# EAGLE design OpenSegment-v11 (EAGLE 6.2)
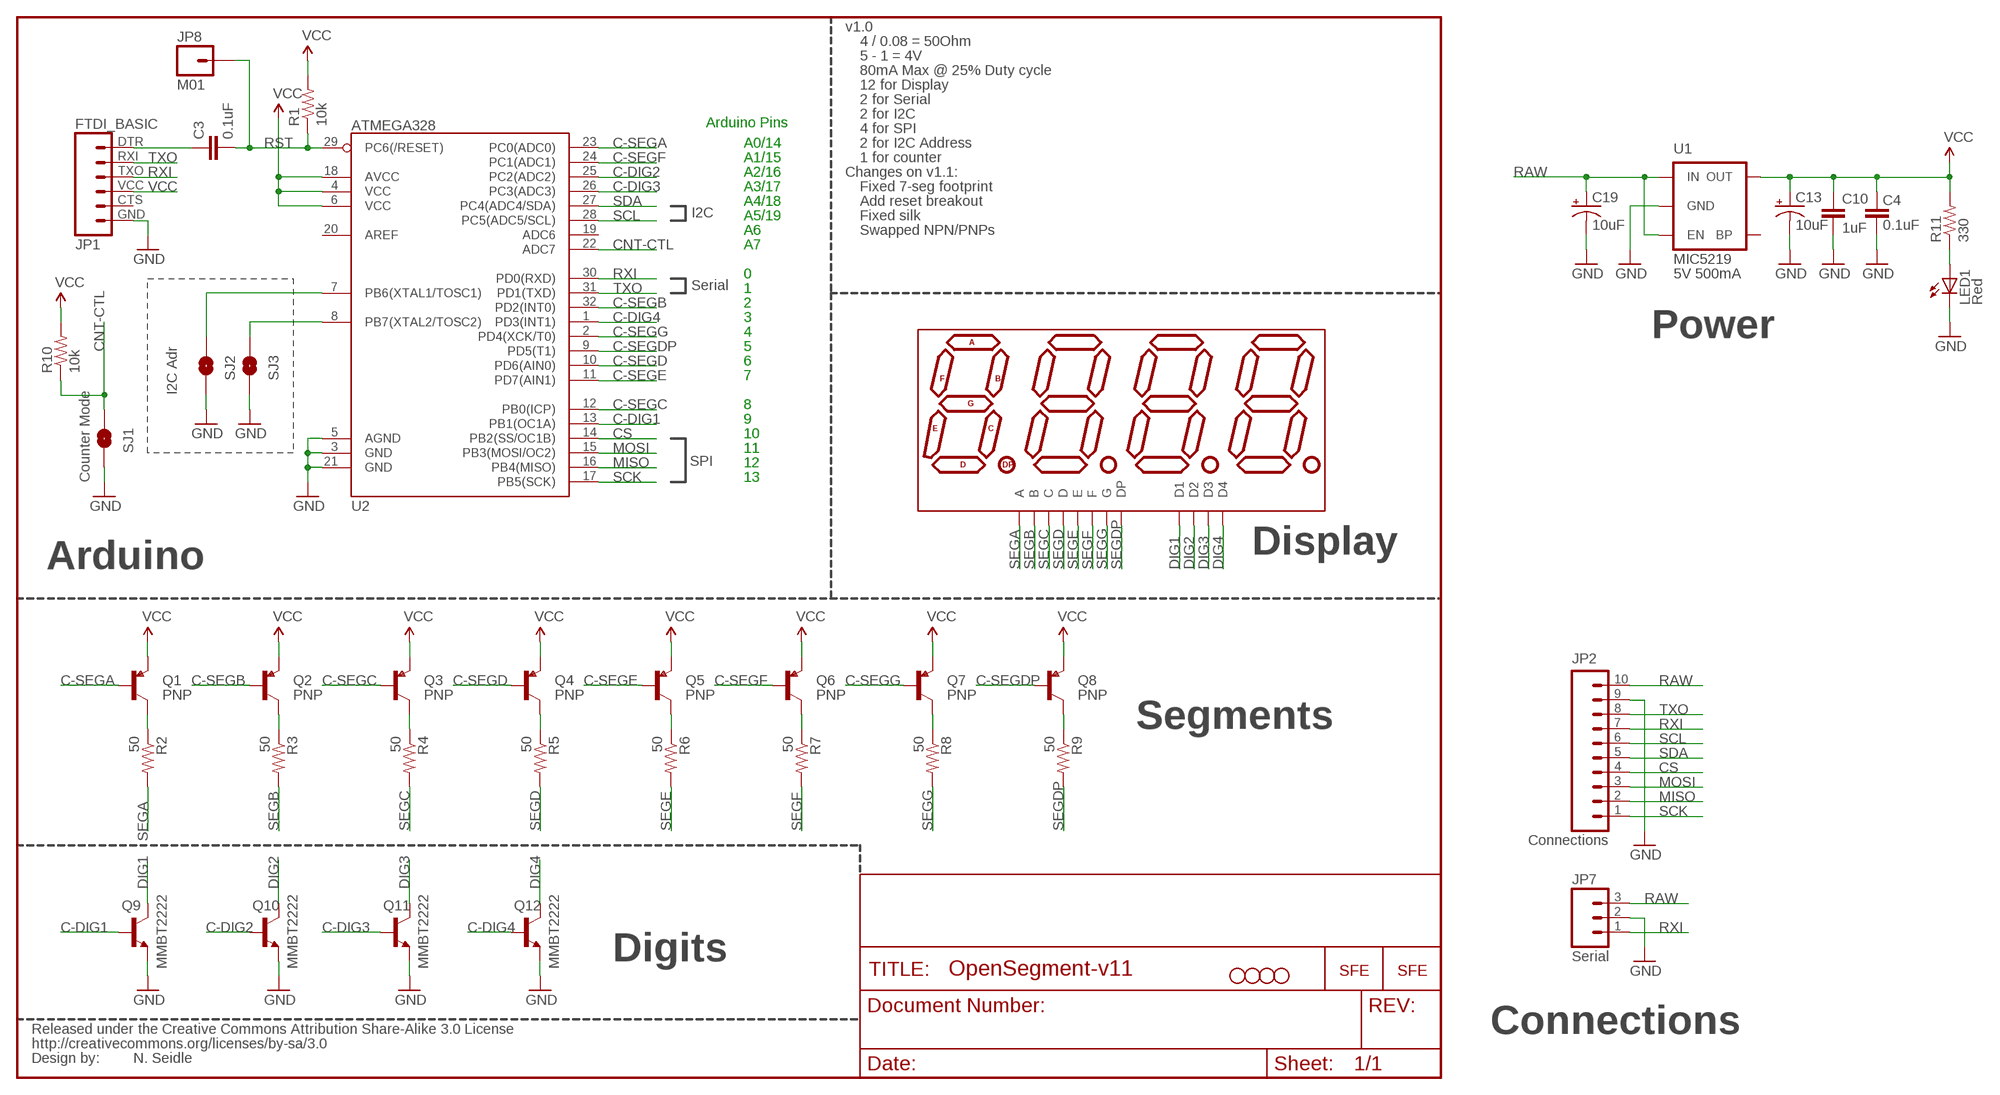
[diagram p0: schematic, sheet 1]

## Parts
C3  0.1uF  CAP0402-CAP  [0402-CAP]
C4  0.1uF  CAP0402-CAP  [0402-CAP]
C10  1uF  CAP0402-CAP  [0402-CAP]
C13  10uF  CAP_POL1206  [EIA3216]
C19  10uF  CAP_POL1206  [EIA3216]
JP1  FTDI_BASIC  FTDI_BASICPTH  [FTDI_BASIC]
JP2  Connections  M10"  [1X10]
JP3  STAND-OFF  [STAND-OFF]
JP4  STAND-OFF  [STAND-OFF]
JP5  STAND-OFF  [STAND-OFF]
JP6  STAND-OFF  [STAND-OFF]
JP7  Serial  M03  [JST-3-SMD]
JP8  M01  M01PTH  [1X01]
LED1  Red  LED0603  [LED-0603]
Q1  PNP  TRANSISTOR_PNPSMD  [SOT23-3]
Q2  PNP  TRANSISTOR_PNPSMD  [SOT23-3]
Q3  PNP  TRANSISTOR_PNPSMD  [SOT23-3]
Q4  PNP  TRANSISTOR_PNPSMD  [SOT23-3]
Q5  PNP  TRANSISTOR_PNPSMD  [SOT23-3]
Q6  PNP  TRANSISTOR_PNPSMD  [SOT23-3]
Q7  PNP  TRANSISTOR_PNPSMD  [SOT23-3]
Q8  PNP  TRANSISTOR_PNPSMD  [SOT23-3]
Q9  MMBT2222  TRANSISTOR_NPNSOT23-3  [SOT23-3]
Q10  MMBT2222  TRANSISTOR_NPNSOT23-3  [SOT23-3]
Q11  MMBT2222  TRANSISTOR_NPNSOT23-3  [SOT23-3]
Q12  MMBT2222  TRANSISTOR_NPNSOT23-3  [SOT23-3]
R1  10k  RESISTOR0402-RES  [0402-RES]
R2  50  RESISTOR0402-RES  [0402-RES]
R3  50  RESISTOR0402-RES  [0402-RES]
R4  50  RESISTOR0402-RES  [0402-RES]
R5  50  RESISTOR0402-RES  [0402-RES]
R6  50  RESISTOR0402-RES  [0402-RES]
R7  50  RESISTOR0402-RES  [0402-RES]
R8  50  RESISTOR0402-RES  [0402-RES]
R9  50  RESISTOR0402-RES  [0402-RES]
R10  10k  RESISTOR0402-RES  [0402-RES]
R11  330  RESISTOR0402-RES  [0402-RES]
SJ1  Counter Ctl  SOLDERJUMPERNO  [SJ_2S-NO]
SJ2  Counter Ctl  SOLDERJUMPERNO  [SJ_2S-NO]
SJ3  Counter Ctl  SOLDERJUMPERNO  [SJ_2S-NO]
U1  MIC5219  V_REG_LDOSMD  [SOT23-5]
U2  ATMEGA328  ATMEGA168  [TQFP32-08]
U3  7-SEGMENT-4DIGIT-COUNTERPTH  [7-SEGMENT-4DIGIT-COUNTER]
U$2  LOGO-SFESK  [SFE-LOGO-FLAME]
U$3  CREATIVE_COMMONS  [CREATIVE_COMMONS]
U$7  LOGO-SFENW2  [SFE-NEW-WEB]

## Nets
C-DIG1: Q9.1(B) U2.13(PB1(OC1A))
C-DIG2: Q10.1(B) U2.25(PC2(ADC2))
C-DIG3: Q11.1(B) U2.26(PC3(ADC3))
C-DIG4: Q12.1(B) U2.1(PD3(INT1))
C-SEGA: Q1.1(B) U2.23(PC0(ADC0))
C-SEGB: Q2.1(B) U2.32(PD2(INT0))
C-SEGC: Q3.1(B) U2.12(PB0(ICP))
C-SEGD: Q4.1(B) U2.10(PD6(AIN0))
C-SEGDP: Q8.1(B) U2.9(PD5(T1))
C-SEGE: Q5.1(B) U2.11(PD7(AIN1))
C-SEGF: Q6.1(B) U2.24(PC1(ADC1))
C-SEGG: Q7.1(B) U2.2(PD4(XCK/T0))
CNT-CTL: R10.1 SJ1.1 U2.22(ADC7)
CS: JP2.4 U2.14(PB2(SS/OC1B))
DIG1: Q9.3(C) U3.12(D1)
DIG2: Q10.3(C) U3.9(D2)
DIG3: Q11.3(C) U3.8(D3)
DIG4: Q12.3(C) U3.6(D4)
GND: C4.1 C10.2 C13.C(-) C19.C(-) JP1.GND JP2.9 JP7.2 LED1.C Q9.2(E) Q10.2(E) Q11.2(E) Q12.2(E) SJ1.2 SJ2.2 SJ3.2 U1.2(GND) U2.3(GND) U2.5(AGND) U2.21(GND)
MISO: JP2.2 U2.16(PB4(MISO))
MOSI: JP2.3 U2.15(PB3(MOSI/OC2))
N$1: Q1.3(C) R2.1
N$2: SJ3.1 U2.8(PB7(XTAL2/TOSC2))
N$3: C3.1 JP1.DTR
N$4: Q2.3(C) R3.1
N$5: Q3.3(C) R4.1
N$6: Q4.3(C) R5.1
N$7: Q5.3(C) R6.1
N$8: Q6.3(C) R7.1
N$9: Q7.3(C) R8.1
N$10: Q8.3(C) R9.1
N$18: SJ2.1 U2.7(PB6(XTAL1/TOSC1))
N$38: LED1.A R11.1
RAW [vcc]: C19.A(+) JP2.10 JP7.3 U1.1(IN) U1.3(EN)
RST: C3.2 JP8.1 R1.1 U2.29(PC6(/RESET))
RXI: JP1.TXO JP2.7 JP7.1 U2.30(PD0(RXD))
SCK: JP2.1 U2.17(PB5(SCK))
SCL: JP2.6 U2.28(PC5(ADC5/SCL))
SDA: JP2.5 U2.27(PC4(ADC4/SDA))
SEGA: R2.2 U3.11(A)
SEGB: R3.2 U3.7(B)
SEGC: R4.2 U3.4(C)
SEGD: R5.2 U3.2(D)
SEGDP: R9.2 U3.3(DP)
SEGE: R6.2 U3.1(E)
SEGF: R7.2 U3.10(F)
SEGG: R8.2 U3.5(G)
TXO: JP1.RXI JP2.8 U2.31(PD1(TXD))
VCC: C4.2 C10.1 C13.A(+) JP1.VCC Q1.2(E) Q2.2(E) Q3.2(E) Q4.2(E) Q5.2(E) Q6.2(E) Q7.2(E) Q8.2(E) R1.2 R10.2 R11.2 U1.5(OUT) U2.4(VCC) U2.6(VCC) U2.18(AVCC)
Unconnected: JP1.CTS U1.4(BP) U2.19(ADC6) U2.20(AREF)

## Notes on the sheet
- v1.0
- 4 / 0.08 = 50Ohm
- 5 - 1 = 4V
- 80mA Max @ 25% Duty cycle
- 12 for Display
- 2 for Serial
- 2 for I2C
- Arduino Pins
- 4 for SPI
- A0/14 | 2 for I2C Address
- A1/15 | 1 for counter
- A2/16 | Changes on v1.1:
- A3/17 | Fixed 7-seg footprint
- A4/18 | Add reset breakout
- I2C | A5/19 | Fixed silk
- A6 | Swapped NPN/PNPs
- A7
- 0 | 5V 500mA
- Serial | 1
- 2
- 3
- 4 | Power
- 5
- 6
- 7
- I2C Adr
- 8
- 9
- 10
- 11
- SPI | 12
- Counter Mode | 13
- Display
- Arduino
- Segments
- Digits
- Connections
- N. Seidle

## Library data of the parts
C3 C4 C10 = SparkFun:CAP: Capacitor
C13 C19 = SparkFun:CAP_POL: Capacitor Polarized
JP1 = SparkFun:FTDI_BASIC: FTDI Basic: 3.3V and 5V
JP2 = SparkFun-Connectors:M10: Header 10 Standard 10-pin 0.1" header. Use with straight break away headers (SKU : PRT-00116), right angle break away headers (PRT-00553), swiss pins (PRT-00743), machine pins (PRT-00117), and female headers (PRT-00115).
JP3-JP6 = SparkFun-Electromechanical:STAND-OFF: #4 Stand Off
JP7 = SparkFun-Connectors:M03: Header 3 Standard 3-pin 0.1" header. Use with straight break away headers (SKU : PRT-00116), right angle break away headers (PRT-00553), swiss pins (PRT-00743), machine pins (PRT-00117), and female headers (PRT-00115). Molex polarized connector foot print use with SKU : PRT-08232 with associated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
JP8 = SparkFun-Connectors:M01: Header 1
LED1 = SparkFun:LED: LEDs
Q1-Q8 = SparkFun-DiscreteSemi:TRANSISTOR_PNP: Generic PNP BJT. Double check pinouts against datasheets- not all devices are the same!
Q9-Q12 = SparkFun-DiscreteSemi:TRANSISTOR_NPN: Generic NPN BJT. MMBT2222 is the common NPN we use. Double check against datasheet- not all devices are the same!
R1-R11 = SparkFun:RESISTOR: Resistor
SJ1-SJ3 = SparkFun-Passives:SOLDERJUMPER: Solder Jumper
U1 = SparkFun:V_REG_LDO: Voltage Regulator LDO Standard 150mA LDO voltage regulator in SOT-23 layout. Micrel part MIC5205. BP (by-pass) pin is used to lower output noise with 470pF cap.
U2 = SparkFun-DigitalIC:ATMEGA168: Atmel 32-pin 8-bit micro, 16k flash.
U3 = SparkFun-Displays:7-SEGMENT-4DIGIT-COUNTER
U$2 U$7 = SparkFun:LOGO-SFE: Spark Fun Electronics PCB Logo
U$3 = SparkFun:CREATIVE_COMMONS

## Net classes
0 default: width 0.203 mm

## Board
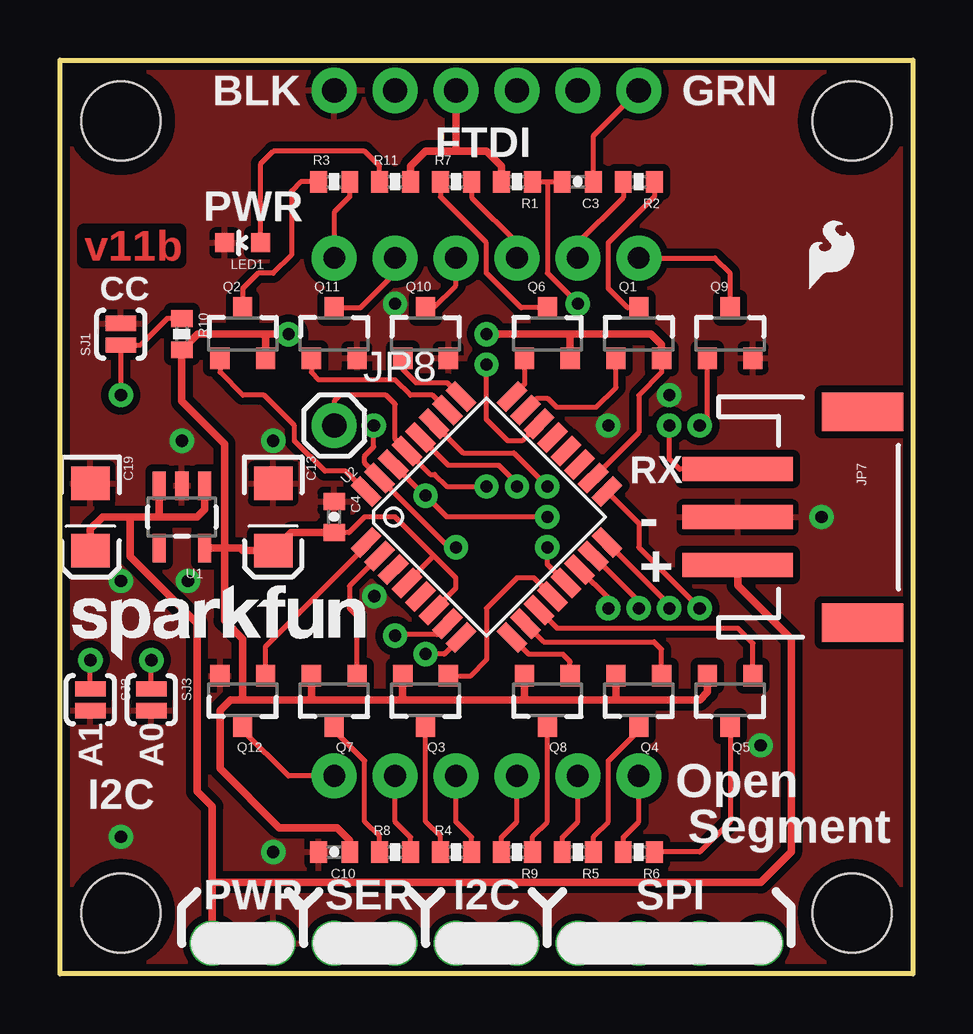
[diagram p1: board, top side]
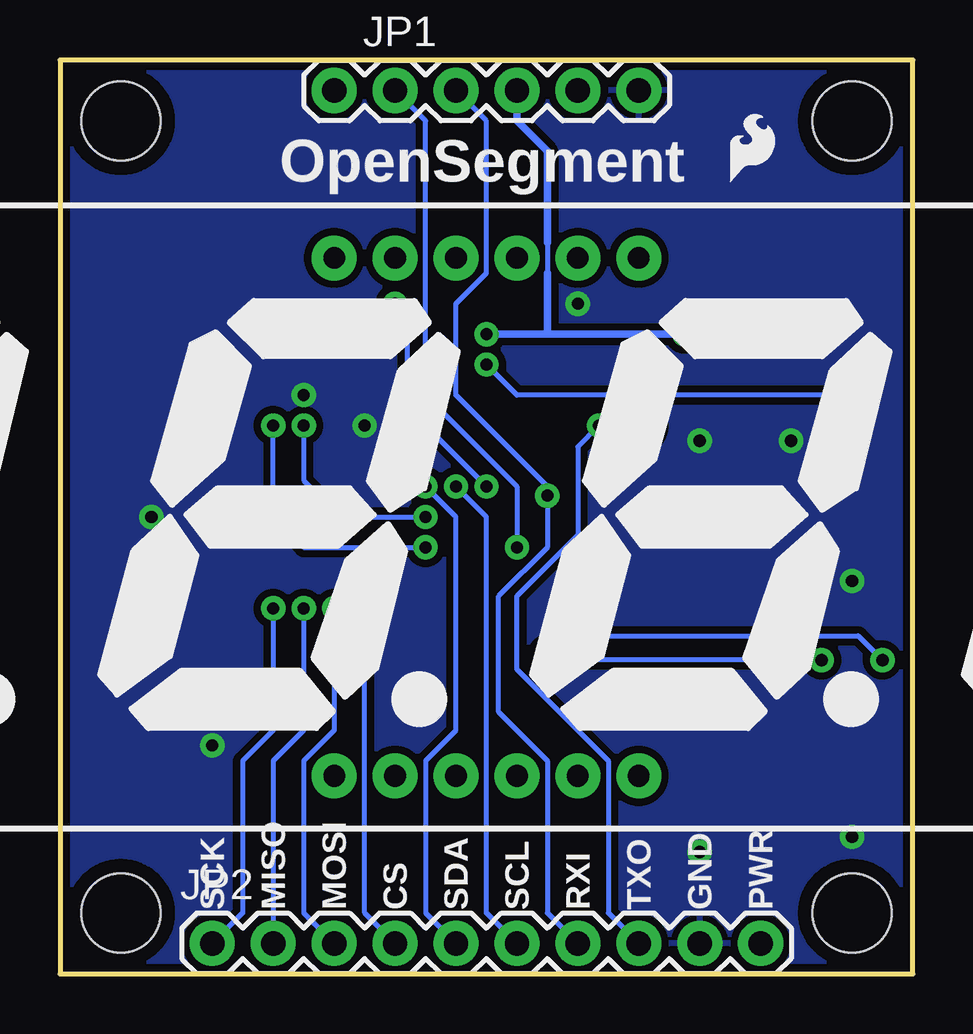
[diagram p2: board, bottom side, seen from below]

Size 35.56 x 38.1 mm. Coordinates in mm from the lower left corner, seen from the top.
Outline: 35.56,38.1 35.56,0 0,0 0,38.1 35.56,38.1
Copper layers (1*16): Top 0.035mm / dielectric 1.5mm / Bottom 0.035mm
Design rules: minimum track width 8mil, minimum drill 20mil, track to track 8mil, track to pad 8mil, pad to pad 8mil, via to via 8mil, smd to smd 8mil, copper to edge 10mil, drill to drill 8mil, minimum pad ring 12mil, minimum via ring 10mil, stop-mask expansion 4mil, vias tented up to drill 20mil, thermal gap 10mil

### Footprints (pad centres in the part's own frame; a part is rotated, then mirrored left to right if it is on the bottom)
0402-CAP = smd 0.7 x 0.9: 1 -0.65,0; 2 0.65,0
EIA3216 = smd 1.4 x 1.6: A 1.4,0; C -1.4,0
FTDI_BASIC = drill 1.016 pad 1.88: CTS 10.16,0; DTR 0,0; GND 12.7,0; RXI 2.54,0; TXO 5.08,0; VCC 7.62,0
1X10 = drill 1.016 pad 1.88: 1 0,0; 2 2.54,0; 3 5.08,0; 4 7.62,0; 5 10.16,0; 6 12.7,0; 7 15.24,0; 8 17.78,0; 9 20.32,0; 10 22.86,0
STAND-OFF = hole 3.302: 0,0
JST-3-SMD = smd 1 x 4.6: 1 -1.99,-4.77; 2 0.01,-4.77; 3 2.01,-4.77 | smd 1.6 x 3.4: NC1 -4.39,0.43; NC2 4.41,0.43
1X01 = drill 1.016 pad 1.88: 1 0,0
LED-0603 = smd 0.8 x 0.8: A 0,-0.75; C 0,0.75
SOT23-3 = smd 0.8 x 0.9: 1 -0.95,-1; 2 0.95,-1; 3 0,1.1
0402-RES = smd 0.7 x 0.9: 1 -0.65,0; 2 0.65,0
SJ_2S-NO = smd 0.635 x 1.27: 1 -0.45,0; 2 0.45,0
SOT23-5 = smd 0.55 x 1.2: 1 -0.95,-1.3; 2 0,-1.3; 3 0.95,-1.3; 4 0.95,1.3; 5 -0.95,1.3
TQFP32-08 = smd 1.27 x 0.559: 1 -4.293,2.8; 2 -4.293,2; 3 -4.293,1.2; 4 -4.293,0.4; 5 -4.293,-0.4; 6 -4.293,-1.2; 7 -4.293,-2; 8 -4.293,-2.8; 17 4.293,-2.8; 18 4.293,-2; 19 4.293,-1.2; 20 4.293,-0.4; 21 4.293,0.4; 22 4.293,1.2; 23 4.293,2; 24 4.293,2.8 | smd 0.559 x 1.27: 9 -2.8,-4.293; 10 -2,-4.293; 11 -1.2,-4.293; 12 -0.4,-4.293; 13 0.4,-4.293; 14 1.2,-4.293; 15 2,-4.293; 16 2.8,-4.293; 25 2.8,4.293; 26 2,4.293; 27 1.2,4.293; 28 0.4,4.293; 29 -0.4,4.293; 30 -1.2,4.293; 31 -2,4.293; 32 -2.8,4.293
7-SEGMENT-4DIGIT-COUNTER = drill 0.9 pad 1.88: 1 -6.35,-10.795; 2 -3.81,-10.795; 3 -1.27,-10.795; 4 1.27,-10.795; 5 3.81,-10.795; 6 6.35,-10.795; 7 6.35,10.795; 8 3.81,10.795; 9 1.27,10.795; 10 -1.27,10.795; 11 -3.81,10.795; 12 -6.35,10.795

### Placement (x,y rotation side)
C3  21.59,33.02 180 top
C4  11.43,19.05 270 top
C10  11.43,5.08 180 top
C13  8.89,19.05 270 top
C19  1.27,19.05 270 top
JP1  24.13,36.83 0 bottom
JP2  29.21,1.27 0 bottom
JP3  33.02,35.56 0 top
JP4  2.54,35.56 0 top
JP5  33.02,2.54 0 top
JP6  2.54,2.54 0 top
JP7  33.02,19.05 270 top
JP8  11.43,22.86 0 top
LED1  7.62,30.48 90 top
Q1  24.13,26.67 0 top
Q2  7.62,26.67 0 top
Q3  15.24,11.43 180 top
Q4  24.13,11.43 180 top
Q5  27.94,11.43 180 top
Q6  20.32,26.67 0 top
Q7  11.43,11.43 180 top
Q8  20.32,11.43 180 top
Q9  27.94,26.67 0 top
Q10  15.24,26.67 0 top
Q11  11.43,26.67 0 top
Q12  7.62,11.43 180 top
R1  19.05,33.02 180 top
R2  24.13,33.02 180 top
R3  11.43,33.02 0 top
R4  16.51,5.08 0 top
R5  21.59,5.08 180 top
R6  24.13,5.08 180 top
R7  16.51,33.02 0 top
R8  13.97,5.08 0 top
R9  19.05,5.08 180 top
R10  5.08,26.67 270 top
R11  13.97,33.02 0 top
SJ1  2.54,26.67 90 top
SJ2  1.27,11.43 270 top
SJ3  3.81,11.43 270 top
U1  5.08,19.05 180 top
U2  17.78,19.05 45 top
U3  17.78,19.05 0 bottom
U$1  LOGO-SFESK  [SFE-LOGO-FLAME]  7.62,33.02 0 bottom
U$2  31.24,28.58 0 top
U$3  not placed on the board
U$7  0.51,13.08 0 top

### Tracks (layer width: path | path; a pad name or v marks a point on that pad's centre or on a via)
C-DIG1  (via drill 0.51)
  Top 0.203: U2.13 20.32,17.08 v20.32,17.78 | v26.67,22.86 26.99,23.18 Q9.1
  Bottom 0.203: v20.32,17.78 25.4,17.78 26.67,19.05 v26.67,22.86
C-DIG2
  Top 0.203: U2.25 16.15,24.64 14.86,24.64 14.29,25.21 Q10.1
C-DIG3
  Top 0.203: U2.26 15.53,24.13 14.61,24.13 13.97,24.77 10.8,24.77 10.48,25.08 Q11.1
C-DIG4
  Top 0.203: U2.1 12.77,17.84 8.89,13.97 8.57,13.65 Q12.1
C-SEGA
  Top 0.203: U2.23 19.91,24 20.32,24 20.7,23.62 22.35,23.62 23.18,24.45 Q1.1
C-SEGB
  Top 0.203: Q2.1 6.67,25.08 7.62,24.13 8.51,24.13 9.78,22.86 9.78,22.23 11.05,20.96 11.92,20.96 U2.32
C-SEGC
  Top 0.203: U2.12 19.75,16.51 19.05,16.51 17.78,15.24 17.78,13.08 17.13,12.43 Q3.1
C-SEGD
  Top 0.203: U2.10 20.16,13.84 24.77,13.84 25.08,13.53 Q4.1
C-SEGDP
  Top 0.203: U2.9 19.54,13.34 20.96,13.34 21.27,13.02 Q8.1
C-SEGE
  Top 0.203: U2.11 20.72,14.41 28.26,14.41 28.89,13.78 Q5.1
C-SEGF
  Top 0.203: U2.24 19.37,24.6 Q6.1
C-SEGG
  Top 0.203: U2.2 12.07,16.16 12.07,15.24 12.38,14.93 Q7.1
CNT-CTL  (via drill 0.51)
  Top 0.203: U2.22 19.26,22.23 18.67,22.23 17.78,23.11 v17.78,25.4 | v2.54,24.13 SJ1.1 3.36,26.22 4.46,27.32 R10.1
  Bottom 0.203: v2.54,24.13 16.51,24.13 v17.78,25.4
CS  (via drill 0.51)
  Top 0.203: U2.14 22.86,15.67 v22.86,15.24
  Bottom 0.203: v22.86,15.24 22.86,2.54 JP2.4
DIG1
  Top 0.203: Q9.3 27.94,29.21 27.3,29.84 U3.12
DIG2
  Top 0.203: Q10.3 15.58,27.77 16.51,28.7 U3.9
DIG3
  Top 0.203: Q11.3 12.53,27.77 13.97,29.21 U3.8
DIG4
  Top 0.203: Q12.3 7.62,10.16 9.53,8.26 U3.6
GND  (via drill 0.51)
  other vias: 25.4,24.13 22.86,22.86 31.75,19.05 29.21,9.53 2.54,5.71 8.89,5.08 13.11,15.75 8.89,22.23 5.33,16.38 2.54,16.38 13.97,27.94 5.08,22.23
  pour Top (isolate 0.305): 0,0 0,38.1 35.56,38.1 35.56,0
  pour Bottom (isolate 0.305): 0,0 0,38.1 35.56,38.1 35.56,0
MISO  (via drill 0.51)
  Top 0.203: U2.16 25.4,15.39 v25.4,15.24
  Bottom 0.203: v25.4,15.24 25.4,10.16 26.67,8.89 JP2.2
MOSI  (via drill 0.51)
  Top 0.203: U2.15 24.13,15.53 v24.13,15.24
  Bottom 0.203: v24.13,15.24 24.13,10.16 25.4,8.89 25.4,2.54 JP2.3
N$1
  Top 0.203: Q1.3 23.66,27.77 22.86,28.58 22.86,30.48 24.78,32.4 R2.1
N$2  (via drill 0.51)
  Top 0.203: SJ3.1 v3.81,13.08 | U2.8 16.03,13.34 v15.24,13.34
  Bottom 0.203: v3.81,13.08 14.99,13.08 v15.24,13.34
N$3
  Top 0.203: C3.1 22.24,34.94 JP1.DTR
N$4
  Top 0.203: R3.1 10.03,33.02 9.65,32.64 9.65,29.97 8.89,29.21 8.26,29.21 7.62,28.58 Q2.3
N$5
  Top 0.203: R4.1 15.86,5.73 15.24,6.35 Q3.3
N$6
  Top 0.203: R5.1 22.24,5.73 22.86,6.35 22.86,8.89 24.13,10.16 Q4.3
N$7
  Top 0.203: Q5.3 27.94,6.35 26.67,5.08 R6.1
N$8
  Top 0.203: Q6.3 19.22,27.77 17.78,29.21 17.78,30.48 15.86,32.4 R7.1
N$9
  Top 0.203: R8.1 13.32,5.73 12.7,6.35 12.7,8.89 11.43,10.16 Q7.3
N$10
  Top 0.203: R9.1 19.7,5.73 20.32,6.35 Q8.3
N$18  (via drill 0.51)
  Top 0.203: SJ2.1 v1.27,13.08 | U2.7 15.71,14.15 14.02,14.15 v13.97,14.1
  Bottom 0.203: v13.97,14.1 2.29,14.1 v1.27,13.08
N$38
  Top 0.203: R11.1 13.32,33.67 12.7,34.29 8.89,34.29 8.37,33.77 LED1.A
RAW
  Top 0.305: 6.35,3.81 6.35,6.99 5.72,7.62 5.72,14.61 2.92,17.4 2.92,19.05 | U1.1 6.03,19.37 5.72,19.05 4.19,19.05 | 4.19,19.05 2.92,19.05 | 2.92,19.05 1.78,19.05 1.27,18.54 C19.A | U1.3 4.13,19.11 4.19,19.05 | JP7.3 28.25,16.2 30.48,13.97 30.48,5.08 29.21,3.81 6.35,3.81 | 6.35,3.81 JP2.10
RST  (via drill 0.51)
  Top 0.203: R1.1 20.32,33.02 | 20.32,33.02 C3.2 | 20.32,33.02 20.32,29.21 v21.59,27.94 | v17.78,20.32 16.13,20.32 15.62,20.83 15.44,20.83 U2.29 13.97,22.29 13.97,23.75 13.59,24.13 11.68,24.13 11.43,23.88 JP8.1
  Bottom 0.203: v17.78,20.32 21.08,23.62 21.08,26.67 21.59,27.18 v21.59,27.94
RXI  (via drill 0.51)
  Top 0.203: U2.30 15.19,19.94 v15.24,19.94 16.13,19.05 v20.32,19.05 | JP7.1 25.82,21.04 25.4,21.46 v25.4,22.86
  Bottom 0.203: v20.32,19.05 23.88,19.05 25.4,20.57 v25.4,22.86 | JP2.7 15.24,2.54 15.24,8.89 17.27,10.92 17.27,15.75 15.24,17.78 v15.24,19.94 15.24,20.32 19.05,24.13 19.05,27.94 17.78,29.21 17.78,35.56 JP1.TXO
SCK  (via drill 0.51)
  Top 0.203: U2.17 24.13,18.77 24.13,17.78 v26.67,15.24
  Bottom 0.203: v26.67,15.24 26.67,10.16 27.94,8.89 27.94,2.54 JP2.1
SCL  (via drill 0.51)
  Top 0.203: U2.28 16.19,21.21 18.29,21.21 19.05,20.45 v19.05,20.32
  Bottom 0.203: v19.05,20.32 17.78,19.05 17.78,2.54 JP2.6
SDA  (via drill 0.51)
  Top 0.203: U2.27 16.81,21.72 18.92,21.72 v20.32,20.32
  Bottom 0.203: v20.32,20.32 19.05,19.05 19.05,10.16 20.32,8.89 20.32,2.54 JP2.5
SEGA
  Top 0.203: U3.11 21.59,30.48 23.48,32.37 R2.2
SEGB
  Top 0.203: R3.2 12.08,32.4 11.43,31.75 U3.7
SEGC
  Top 0.203: R4.2 17.16,5.7 16.51,6.35 U3.4
SEGD
  Top 0.203: R5.2 20.94,5.7 21.59,6.35 U3.2
SEGDP
  Top 0.203: R9.2 18.4,5.7 19.05,6.35 U3.3
SEGE
  Top 0.203: R6.2 23.48,5.7 24.13,6.35 U3.1
SEGF
  Top 0.203: R7.2 17.16,32.37 19.05,30.48 U3.10
SEGG
  Top 0.203: R8.2 14.62,5.7 13.97,6.35 U3.5
TXO  (via drill 0.51)
  Top 0.203: v16.51,17.78 16.22,17.78 U2.31 12.7,21.3 12.7,21.59 13.08,21.97 v13.08,22.86
  Bottom 0.203: v16.51,17.78 16.51,20.32 20.32,24.13 20.32,35.56 JP1.RXI | JP2.8 12.7,2.54 12.7,8.89 16.51,12.7 16.51,15.75 13.97,18.29 13.97,21.97 v13.08,22.86
VCC  (via drill 0.51)
  Top 0.203: U2.18 24.13,22.57 24.13,24.13 25.08,25.08 Q1.2 | U2.4 15.56,17.39 15.56,17.46 | C4.2 12.05,18.4 12.7,19.05 13.97,19.05 15.56,17.46 | U2.6 16.51,16.08 16.51,16.51 15.56,17.46
  Top 0.305: 21.21,26.67 24.64,26.67 25.08,26.23 Q1.2 | R1.2 18.4,33.67 17.78,34.29 16.51,34.29 | R11.2 14.62,33.67 15.24,34.29 16.51,34.29 | 6.86,17.75 6.86,22.1 5.08,23.88 R10.2 5.73,26.67 8.51,26.67 | U1.5 6.86,17.75 | 6.86,17.75 7.52,17.75 7.62,17.65 C13.A 9.64,18.4 C4.2 | C10.1 12.08,5.57 11.56,6.1 9.14,6.1 6.67,8.57 6.67,10.99 7.11,11.43 7.62,11.43 | 16.51,34.29 JP1.VCC | v9.53,26.67 8.51,26.67 | Q2.2 8.57,26.61 8.51,26.67 | Q6.2 21.27,26.61 21.21,26.67 | Q5.2 26.99,11.75 26.67,11.43 23.11,11.43 | 23.11,11.43 19.43,11.43 | 19.43,11.43 14.22,11.43 | 14.22,11.43 10.54,11.43 | 10.54,11.43 7.62,11.43 | Q7.2 10.48,11.49 10.54,11.43 | Q3.2 14.29,11.5 14.22,11.43 | Q8.2 19.37,11.49 19.43,11.43 | Q4.2 23.18,11.5 23.11,11.43 | 7.62,11.43 7.62,13.97 6.86,14.73 6.86,17.75 | v17.78,26.67 21.21,26.67
  Bottom 0.203: 15.24,30.48 15.24,29.21
  Bottom 0.305: JP1.VCC 16.51,35.56 15.24,34.29 15.24,30.48 | v17.78,26.67 15.24,26.67 | 15.24,26.67 v9.53,26.67 | 15.24,29.21 15.24,26.67

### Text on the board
Top: v11b
tPlace: BLK | GRN | FTDI | PWR | CC | RX | - | + | A1 | A0 | I2C | Open | Segment | PWR | SER | I2C | SPI | N. Seidle
bPlace: OpenSegment | PWR | GND | TXO | RXI | SCL | SDA | CS | MOSI | MISO | SCK

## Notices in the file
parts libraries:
SparkFun: Released under the Creative Commons Attribution Share-Alike 3.0 License
SparkFun: http://creativecommons.org/licenses/by-sa/3.0
SparkFun-Displays: Licensing: CC v3.0 Share-Alike You are welcome to use this library for commercial purposes.
